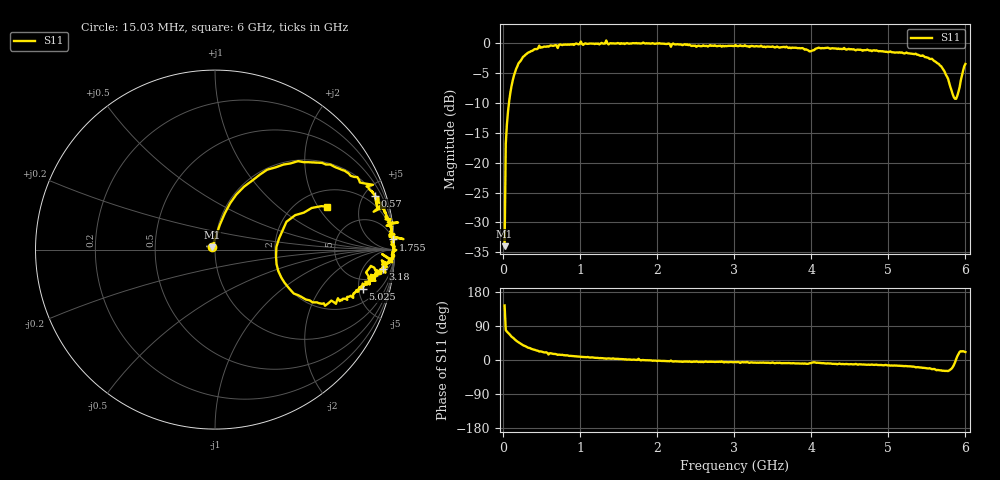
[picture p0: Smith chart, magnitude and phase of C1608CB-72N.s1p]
!	Network	Analyzer	HP8753E.07.74:	Oct	30	2002	Serial	No.	JP38451487
!	Hewlett-Packard
!	7	Sep	2009	9:50:12
!	Frequency	S11
#	HZ	S	RI	R	50
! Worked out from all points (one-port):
!   400 points, 15.03 MHz to 6 GHz, reference 50 ohm
!   lowest |S11| = -34.0 dB at 15.03 MHz (marker M1), VSWR 1.04, Z = 48.4 + j1.14 ohm
!   |S11| at or under -10 dB: start of sweep to 71.9 MHz
!   S11 on the Smith chart (normalised r, x): 15.03 MHz: 0.97, +0.02; 570 MHz: 1.14, +5.86; 1.755 GHz: 3, +35; 3.18 GHz: 7, -14; 5.025 GHz: 3.46, -5.52; 6 GHz: 2.79, +2.42
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1.502992e7  -0.0162 0.0118
3.002985e7  0.0277 0.14
6.00297e7  0.0842 0.258
1.200294e8  0.249 0.417
1.95029e8  0.463 0.493
3.150284e8  0.694 0.45
4.650277e8  0.88 0.361
5.700272e8  0.89 0.301
5.850271e8  0.904 0.233
7.650262e8  0.934 0.229
1.245024e9  0.971 0.0813
1.335023e9  1.05 0.0584
1.365023e9  0.972 0.0722
1.515022e9  0.983 0.0433
1.755021e9  0.994 0.0565
1.785021e9  0.991 -0.0165
2.265019e9  0.976 -0.0653
3.015015e9  0.958 -0.0952
3.180014e9  0.934 -0.107
3.765011e9  0.904 -0.132
4.515007e9  0.874 -0.167
5.025005e9  0.823 -0.219
5.265004e9  0.786 -0.235
5.565002e9  0.674 -0.302
5.730001e9  0.506 -0.278
5.880001e9  0.342 0.0143
5.94e9  0.447 0.192
6e9  0.625 0.239
